DATA_BLOCK DB97
TITLE =

AUTHOR:INA
FAMILY:StateMac
NAME:nb
VERSION:00.00


    FB97


BEGIN
       Write:=FALSE
       NodeID:=B#16#00
       Done:=FALSE
       Err:=FALSE
       ErrNo:=L#0
       xEdgeMerker:=FALSE
       xEdgeFlag:=FALSE
       xStep:=0
       xSwitchOnDisable:=W#16#0000

END_DATA_BLOCK
